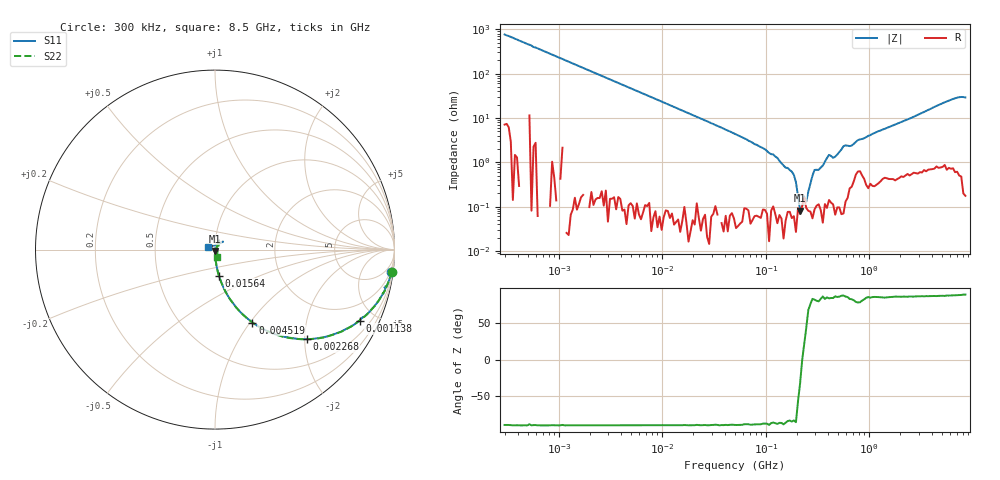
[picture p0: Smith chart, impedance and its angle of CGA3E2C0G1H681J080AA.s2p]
! S-parameter Generated by TDK Corporation
! Copyright(C) 2015 TDK Corporation.
! All Rights Reserved.
! TDK P/N: CGA3E2C0G1H681J080AA (Multilayer Ceramic Chip Capacitors)
! Property: C=680pF
! Size(LxWxT): 1.6x0.8x0.8mm, 0.063x0.031x0.031inches
! Model Type: s2p (Touchstone File Format Version 1.0)
! Frequency: DC=Yes Start=0.3MHz Stop=8500MHz 225points Log-sweep
! Note:
! Model Generated on Jun. 23, 2015
! Hash(MD5):
! Port Assignments:
!  1 ---| |--- 2
! Applicable Conditions:
!  Temperature = 25 degC
!  DC Bias Voltage = 0 V
!  Small Signal Operation
! Terms and conditions regarding TDK Simulation Models
! (1)This simulation model is being provided solely for informational purposes. Please refer to the specifications of the products in terms of detailed characteristics of such products.
! (2)In no event shall TDK Corporation of any of its subsidiaries be liable for any loss or damage arising, directly or indirectly,
!  From any information contained in this simulation model, including, but not limited to loss or damages arising from any inaccuracies, omissions or errors in connection with such information.
! (3)Any and all copyrights on this simulation model are owned by TDK Corporation.
!  Duplication or redistribution of this simulation model without prior written permission from TDK Corporation is prohibited.
! (4)This simulation model is subject to any modification or change without any prior notice.
! (5)Neither TDK Corporation nor any of its subsidiaries shall make any warranty, express or implied,
!  Including but not limited to the correctness, implied warranties of merchantability and fitness for a particular purpose with respect to this simulation models.
! (6)The use of this simulation model shall be deemed to have consented to the terms and conditions hereof.
# MHz S MA R 50
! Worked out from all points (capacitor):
!   224 points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, 300 kHz to 8.5 GHz, reference 50 ohm
!   read as one part in series: C = 686 pF near 314.1 kHz
!   lowest |Z| = 81.5 mohm at 214.9 MHz (marker M1)
!   series resonance near 225.2 MHz, so ESL is about 730 pH
!   S11 on the Smith chart (normalised r, x): 300 kHz: 1, -16; 1.138 MHz: 1.00, -4.06; 2.268 MHz: 1.00, -2.05; 4.519 MHz: 1.00, -1.03; 15.64 MHz: 1.00, -0.30; 8.5 GHz: 0.92, +0.02
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0.3  0.9904 -7.2  0.1296 82.3  0.1299 83.1  0.9915 -7.2
1.137941  0.8976 -26.2  0.4403 63.9  0.4396 63.9  0.8975 -26.1
1.72111  0.8027 -36.5  0.5956 53.4  0.5949 53.4  0.8028 -36.6
2.267783  0.7145 -44.3  0.6988 45.6  0.6987 45.6  0.7146 -44.3
4.519427  0.4568 -62.8  0.8895 27.1  0.889 27.1  0.4566 -62.8
9.430415  0.2389 -76.1  0.9709 13.7  0.9703 13.8  0.2385 -76.2
15.63691  0.1466 -81.5  0.989 8.4  0.9884 8.4  0.1466 -81.4
51.67171  0.04421 -86.9  0.9987 2.4  0.9986 2.3  0.04411 -87.6
214.8731  0.007734 -83.6  0.9994 -0.4  0.999 -0.4  0.007149 -88.6
283.1228  0.004082 -80.1  0.9996 -0.8  0.999 -0.8  0.003457 -90.5
373.0505  0.001414 -52.2  0.9979 -1.2  0.9983 -1.2  0.0004725 115.2
428.2171  0.0006822 32.0  0.9975 -1.5  0.9979 -1.5  0.001369 102.3
448.3627  0.001477 2.5  0.9984 -1.4  0.9976 -1.4  0.001926 117.4
564.2308  0.002689 57.9  0.9981 -2.5  0.9992 -2.4  0.004967 101.0
710.042  0.007248 44.5  0.9952 -2.7  0.9964 -2.6  0.005144 68.6
935.5712  0.003489 62.8  0.9972 -4.1  0.9965 -4.1  0.005315 26.1
1551.304  0.005648 64.7  0.9944 -6.9  0.9954 -6.8  0.006742 34.8
2572.272  0.007971 57.7  0.9936 -11.3  0.9932 -11.2  0.008784 35.4
6161.135  0.06094 45.7  0.9884 -27.2  0.9881 -27.0  0.05851 68.8
7404.957  0.05433 47.3  0.9905 -32.4  0.9876 -32.3  0.05015 63.7
8118.083  0.02379 93.8  0.9916 -35.3  0.9899 -35.1  0.01687 19.2
8500  0.04075 162.7  0.9897 -37.0  0.9904 -36.8  0.04114 -74.4
